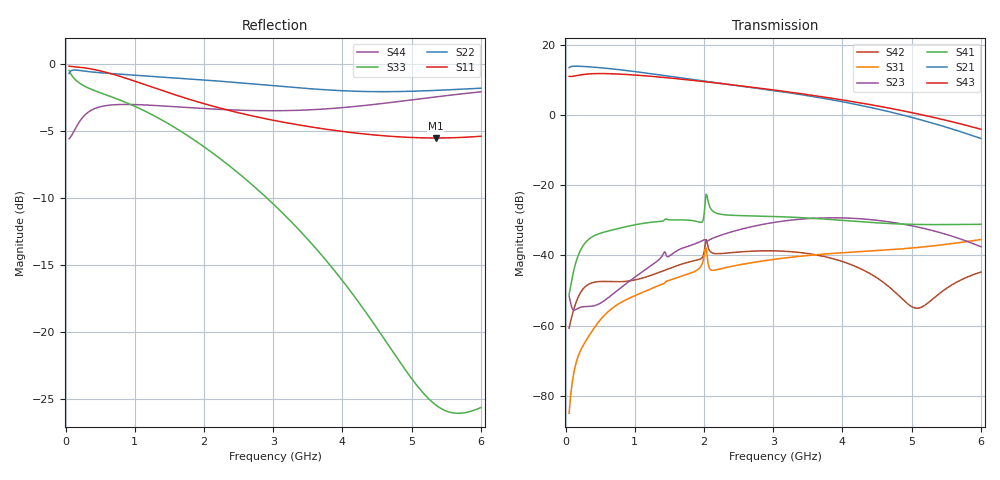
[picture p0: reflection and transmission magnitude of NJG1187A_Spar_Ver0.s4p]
! Created Wed Mar 10 19:53:37 2021
# hz S ma R 50
! 4 Port Network Data from SP11.SP block
! freq  magS11  angS11  magS12  angS12  magS13  angS13  magS14  angS14
!  magS21  angS21  magS22  angS22  magS23  angS23  magS24  angS24
!  magS31  angS31  magS32  angS32  magS33  angS33  magS34  angS34
!  magS41  angS41  magS42  angS42  magS43  angS43  magS44  angS44
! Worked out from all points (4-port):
!   596 points, 50 MHz to 6 GHz, reference 50 ohm
!   strongest paths, dB at 50 MHz, 1.54 GHz, 3.03 GHz, 4.52 GHz, 6 GHz:
!     S43: 11.0, 10.4, 7.0, 2.5, -4.1
!     S21: 13.4, 10.9, 6.9, 1.6, -6.7
!     S41: -51.1, -29.9, -28.9, -30.7, -31.1
!     S23: -51.6, -39.6, -30.5, -30.0, -37.5
!     S31: -84.9, -46.8, -41.1, -38.6, -35.5
!     S42: -60.7, -43.4, -38.7, -46.7, -44.7
!   lowest |S11| = -5.5 dB at 5.35 GHz (marker M1), VSWR 3.27, Z = 17.5 - j17.7 ohm
!   |S11| at or under -10 dB: nowhere
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5e7  0.9845 -2.1  0.001699 29.9  0.0001003 -91.9  3.847e-05 74.8
     4.698 -171.4  0.9252 4.0  0.002642 -19.8  0.0007345 130.5
     5.679e-05 143.5  4.892e-05 102.9  0.9488 -6.5  0.007091 81.8
     0.002777 124.8  0.0009256 -124.3  3.533 -178.8  0.5277 0.5
5.6e8  0.9373 -18.5  0.002333 28.0  0.0008686 -128.5  0.0004976 67.0
       4.636 147.6  0.9278 -15.5  0.002282 -83.5  0.001779 148.4
       0.00141 174.0  0.0007685 86.2  0.7733 -24.0  0.03642 41.7
       0.02156 8.2  0.004273 170.7  3.875 158.6  0.6999 -10.4
1.26e9  0.8207 -37.2  0.001954 32.6  0.001302 -152.3  0.0009047 63.4
        3.825 111.1  0.902 -35.1  0.007469 -135.0  0.004319 126.7
        0.003452 93.0  0.001278 81.3  0.6465 -46.5  0.05202 36.5
        0.02988 -43.2  0.005333 132.1  3.527 127.2  0.703 -34.8
1.77e9  0.7428 -48.2  0.0006101 107.2  0.001172 -163.4  0.0009818 63.3
        3.262 88.5  0.8833 -50.5  0.01353 -171.9  0.006145 103.8
        0.005445 40.0  0.001513 101.1  0.5404 -61.8  0.06151 32.4
        0.03186 -87.9  0.00802 104.2  3.153 107.2  0.6898 -51.4
2.96e9  0.6213 -72.2  0.01139 168.7  0.003387 -81.4  0.001533 123.8
        2.256 41.3  0.8342 -94.4  0.029 107.1  0.007047 53.3
        0.008673 -37.8  0.004938 112.8  0.308 -93.6  0.07528 20.4
        0.03603 -171.2  0.01166 45.4  2.293 66.2  0.6713 -92.3
5.35e9  0.5311 -136.7  0.05615 126.1  0.02162 -141.7  0.009215 100.1
        0.7403 -45.4  0.7995 155.0  0.02197 -0.0  0.005895 62.8
        0.01384 -112.4  0.009304 71.8  0.05352 170.0  0.05143 -4.8
        0.02751 95.7  0.002617 49.2  0.9061 0.0  0.7561 176.8
6e9  0.5392 -157.6  0.06891 116.7  0.02733 -158.3  0.01078 83.1
     0.4617 -63.1  0.8146 131.4  0.01331 -15.4  0.008001 45.6
     0.01687 -120.1  0.008417 69.1  0.05241 125.5  0.03233 0.2
     0.02776 80.9  0.005808 44.9  0.6256 -11.7  0.7897 155.4
